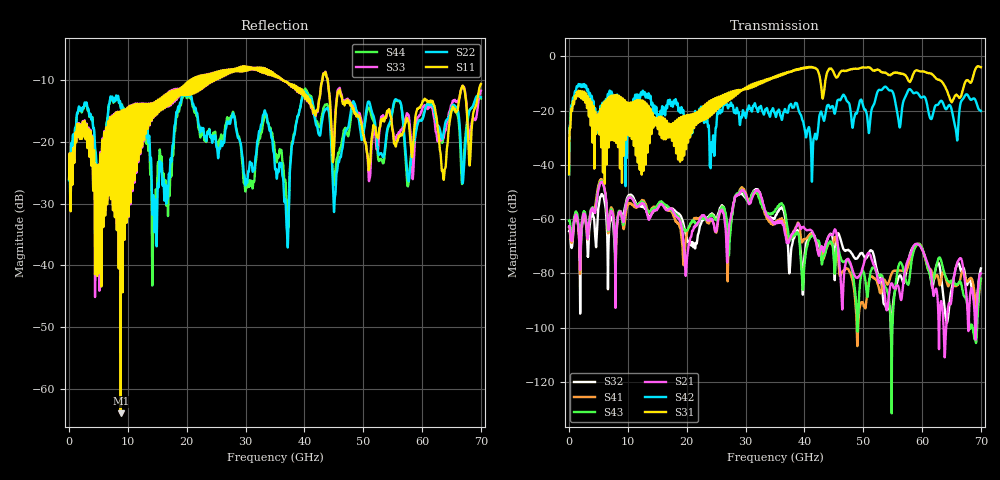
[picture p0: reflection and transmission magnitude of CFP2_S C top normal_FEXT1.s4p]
! AWR Design Environment (8415) Tue Jan 08 13:08:55 2019
! Document = 'CFP2 Channel_S'
! nPorts: 4, nXvals: 7001
# HZ S DB R 50
!Freq DBS11 AngS11 DBS12 AngS12 DBS13 AngS13 DBS14 AngS14
!	DBS21 AngS21 DBS22 AngS22 DBS23 AngS23 DBS24 AngS24
!	DBS31 AngS31 DBS32 AngS32 DBS33 AngS33 DBS34 AngS34
!	DBS41 AngS41 DBS42 AngS42 DBS43 AngS43 DBS44 AngS44
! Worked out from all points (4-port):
!   7000 points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, 10 MHz to 70 GHz, reference 50 ohm
!   strongest paths, dB at 10 MHz, 17.51 GHz, 35.01 GHz, 52.51 GHz, 70 GHz:
!     S31: -43.5, -31.2, -7.4, -5.0, -4.0
!     S42: -43.6, -17.2, -21.2, -12.8, -20.2
!     S21: -62.8, -56.5, -61.8, -82.4, -80.0
!     S43: -60.7, -57.0, -56.9, -80.7, -81.9
!     S41: -63.1, -57.6, -61.7, -84.2, -82.2
!     S32: -64.4, -56.1, -59.3, -80.2, -78.2
!   lowest |S11| = -63.9 dB at 8.78 GHz (marker M1), VSWR 1.00, Z = 50 + j0.058 ohm
!   |S11| at or under -10 dB: start of sweep to 20.78 GHz; 36.27 GHz to 43.07 GHz (6.797 GHz wide, 17.1 % of centre); 43.96 GHz to end of sweep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
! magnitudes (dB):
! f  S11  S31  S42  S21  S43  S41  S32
! 10 MHz  -26.1  -43.5  -43.6  -62.8  -60.7  -63.1  -64.4
! 1.6 GHz  -18.2  -12.7  -10.3  -62.9  -61.3  -63.3  -63.4
! 8.78 GHz  -63.9  -15.7  -17.7  -57.4  -57.4  -57.3  -57.2
! 32 GHz  -8.1  -10.3  -19.9  -49.4  -50.5  -50.7  -49.1
! 37.05 GHz  -10.5  -5.9  -20.6  -68.8  -62.0  -65.9  -65.5
! 40.06 GHz  -12.8  -4.2  -26.9  -63.6  -76.0  -67.5  -72.9
! 70 GHz  -10.7  -4.0  -20.2  -80.0  -81.9  -82.2  -78.2
